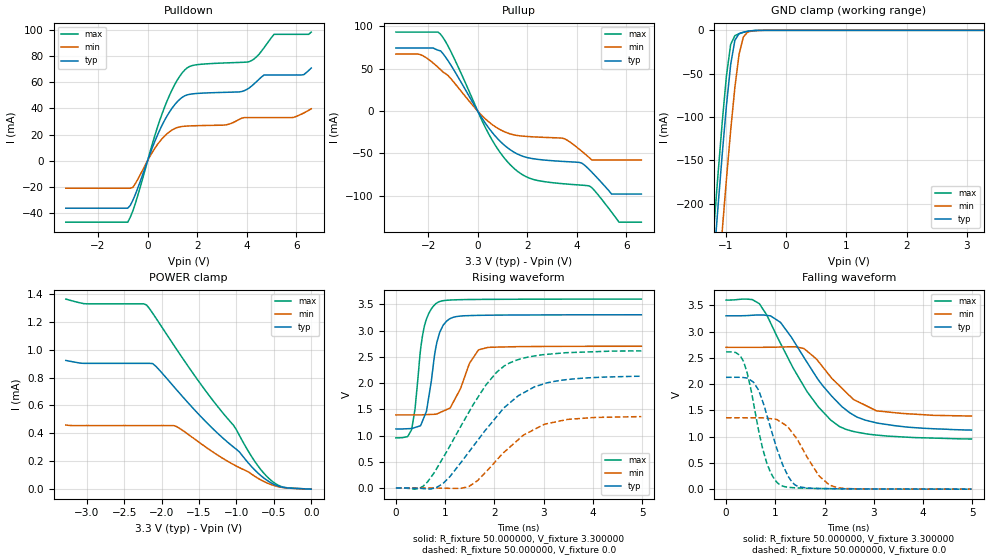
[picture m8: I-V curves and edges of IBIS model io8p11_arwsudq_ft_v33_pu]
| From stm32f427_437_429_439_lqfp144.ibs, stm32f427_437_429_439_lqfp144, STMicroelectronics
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|   Model io8p11_arwsudq_ft_v33_pu
[Model]  io8p11_arwsudq_ft_v33_pu
Model_type I/O
Polarity   Non-Inverting
Enable   Active-Low
Vinl =   0.990000V
Vinh =   2.310000V
Vmeas =  1.650000V
Cref =   30.000000pF
Rref =   100.000000M
Vref =   0.0V
C_comp   2.911600pF   2.826600pF   2.988000pF
[Temperature Range]   25.000000   0.125000k   -40.000000
[Pullup Reference]   3.300000V   2.700000V   3.600000V
[Pulldown Reference]   0.0V   0.0V   0.0V
[POWER Clamp Reference]   3.300000V   2.700000V   3.600000V
[GND Clamp Reference]   0.0V   0.0V   0.0V
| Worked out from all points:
|   slope of the pulldown table from 0 to 0.495 V, typ, clamps not added: 20.9 ohm
|   slope of the pullup table from 0 to 0.495 V, typ, clamps not added: 22.6 ohm
|   GND clamp passes 1 mA (typ) near -0.62 V on its own axis
|   rising waveform, R_fixture 50.000000, V_fixture 3.300000: 20-80 % time 222ps typ, 364ps min, 191ps max; typ from 1.12 V to 3.3 V
|   rising waveform, R_fixture 50.000000, V_fixture 0.0: 20-80 % time 1.15ns typ, 960ps min, 1.02ns max; typ from 0.001 V to 2.13 V
|   falling waveform, R_fixture 50.000000, V_fixture 3.300000: 20-80 % time 1.02ns typ, 835ps min, 1ns max; typ from 3.3 V to 1.12 V
|   falling waveform, R_fixture 50.000000, V_fixture 0.0: 20-80 % time 438ps typ, 539ps min, 360ps max; typ from 2.13 V to 0.001 V
[Pulldown]
|Voltage   I(typ)   I(min)   I(max)
-3.3V     -36.38mA   -21.07mA   -47.09mA
-800mV    -36.38mA   -21.07mA   -47.09mA
-600mV    -30.5mA    -20.54mA   -38.69mA
700mV     31.4mA     19.11mA    41.71mA
1.2V      45.15mA    25.37mA    61.75mA
1.6V      50.35mA    26.5mA     71.06mA
3.1V      52.28mA    27.26mA    74.76mA
4.1V      55.65mA    32.94mA    75.79mA
4.7V      65.59mA    32.94mA    86.49mA
5.1V      65.59mA    32.94mA    96.67mA
6.3V      65.82mA    36.48mA    96.67mA
6.6V      70.87mA    39.69mA    98.38mA
[Pullup]
|Voltage   I(typ)   I(min)   I(max)
-3.3V     74.6mA     67.42mA    93.38mA
-2.3V     74.6mA     66.59mA    93.38mA
-1.5V     71.22mA    49mA       90.81mA
-1V       50.43mA    35.45mA    65.35mA
500mV     -22.06mA   -14mA      -30.03mA
1.6V      -50.64mA   -28.81mA   -70.96mA
3.5V      -59.52mA   -32.65mA   -85.91mA
4.2V      -61.45mA   -47.47mA   -87.45mA
4.5V      -69.09mA   -55.01mA   -88.4mA
5.4V      -98mA      -57.7mA    -119.3mA
5.7V      -98mA      -57.7mA    -131.2mA
6.6V      -98mA      -57.7mA    -131.2mA
[GND_clamp]
|Voltage   I(typ)   I(min)   I(max)
-3.3V     -2.32A     -2.397A    -2.297A
-1.2V     -266.4mA   -356.3mA   -229.4mA
-1.13V    -203.6mA   -293.1mA   -166.3mA
-1.06V    -143.2mA   -231.4mA   -106.2mA
-990mV    -86.95mA   -171.8mA   -52.65mA
-920mV    -39.66mA   -115.8mA   -16.36mA
-850mV    -11.49mA   -65.84mA   -6.11mA
-780mV    -3.834mA   -27.59mA   -3.88mA
-710mV    -2.09mA    -7.753mA   -2.381mA
-640mV    -1.147mA   -2.129mA   -1.22mA
-570mV    -523.9uA   -800uA     -476.8uA
3.28V     0A         0A         0A
[POWER_clamp]
|Voltage   I(typ)   I(min)   I(max)
-3.28V    922.4uA    459.4uA    1.362mA
-3.04V    901.4uA    455.8uA    1.329mA
-2.2V     901.4uA    455.8uA    1.319mA
-2.08V    882.2uA    455.8uA    1.23mA
-1.8V     712.4uA    448.4uA    1.003mA
-1.4V     478.6uA    298uA      696.5uA
-1.04V    302.3uA    176.6uA    458.6uA
-800mV    163uA      108.7uA    236.3uA
-640mV    82.53uA    56.82uA    118.4uA
-520mV    40.35uA    29.6uA     55.89uA
-400mV    15.52uA    13.26uA    18.69uA
0V        0A         0A         0A
[Ramp]
| variable   typ   min   max
dV/dt_r  1.26589/1.14053n   0.80907/0.95560n   1.56202/1.01814n
dV/dt_f  1.28172/1.01183n   0.77460/0.82445n   1.57153/1.00163n
R_load = 50.000000
[Rising Waveform]
R_fixture= 50.000000
V_fixture= 3.300000
V_fixture_min= 2.700000
V_fixture_max= 3.600000
|time   V(typ)   V(min)   V(max)
0s        1.125V     1.393V     955.5mV
320.3ps   1.134V     1.393V     1.119V
390.4ps   1.154V     1.393V     1.526V
500.5ps   1.187V     1.393V     2.639V
620.6ps   1.463V     1.398V     3.219V
850.9ps   2.839V     1.42V      3.536V
1.101ns   3.227V     1.525V     3.581V
1.491ns   3.284V     2.37V      3.59V
1.682ns   3.289V     2.633V     3.592V
4.985ns   3.3V       2.7V       3.599V
[Rising Waveform]
R_fixture= 50.000000
V_fixture= 0.0
V_fixture_min= 0.0
V_fixture_max= 0.0
|time   V(typ)   V(min)   V(max)
0s        1.302mV    1.126mV    1.747mV
550.6ps   -10.04mV   925.7uV    33.51mV
951ps     82.96mV    -2.953mV   566.2mV
1.481ns   685.7mV    27.94mV    1.444V
1.822ns   1.105V     300.8mV    1.955V
2.282ns   1.597V     753.4mV    2.369V
2.593ns   1.814V     1.01V      2.474V
3.023ns   1.99V      1.216V     2.543V
3.483ns   2.067V     1.307V     2.579V
4.985ns   2.129V     1.36V      2.612V
[Falling Waveform]
R_fixture= 50.000000
V_fixture= 3.300000
V_fixture_min= 2.700000
V_fixture_max= 3.600000
|time   V(typ)   V(min)   V(max)
0s        3.3V       2.7V       3.599V
530.5ps   3.31V      2.7V       3.608V
670.7ps   3.316V     2.7V       3.533V
1.101ns   3.178V     2.705V     2.785V
1.582ns   2.509V     2.677V     1.958V
1.872ns   2.084V     2.436V     1.569V
2.312ns   1.611V     1.959V     1.188V
2.583ns   1.415V     1.712V     1.1V
3.053ns   1.263V     1.492V     1.03V
4.985ns   1.125V     1.393V     955.5mV
[Falling Waveform]
R_fixture= 50.000000
V_fixture= 0.0
V_fixture_min= 0.0
V_fixture_max= 0.0
|time   V(typ)   V(min)   V(max)
0s        2.129V     1.36V      2.612V
350.4ps   2.124V     1.359V     2.441V
560.6ps   2.031V     1.359V     1.624V
670.7ps   1.863V     1.358V     1.074V
830.8ps   1.404V     1.35V      490.5mV
1.101ns   591.8mV    1.285V     81.93mV
1.401ns   82.43mV    1.008V     26.92mV
1.882ns   14.19mV    262mV      13.64mV
2.102ns   10.44mV    77.86mV    10.94mV
4.985ns   1.302mV    1.126mV    1.747mV
